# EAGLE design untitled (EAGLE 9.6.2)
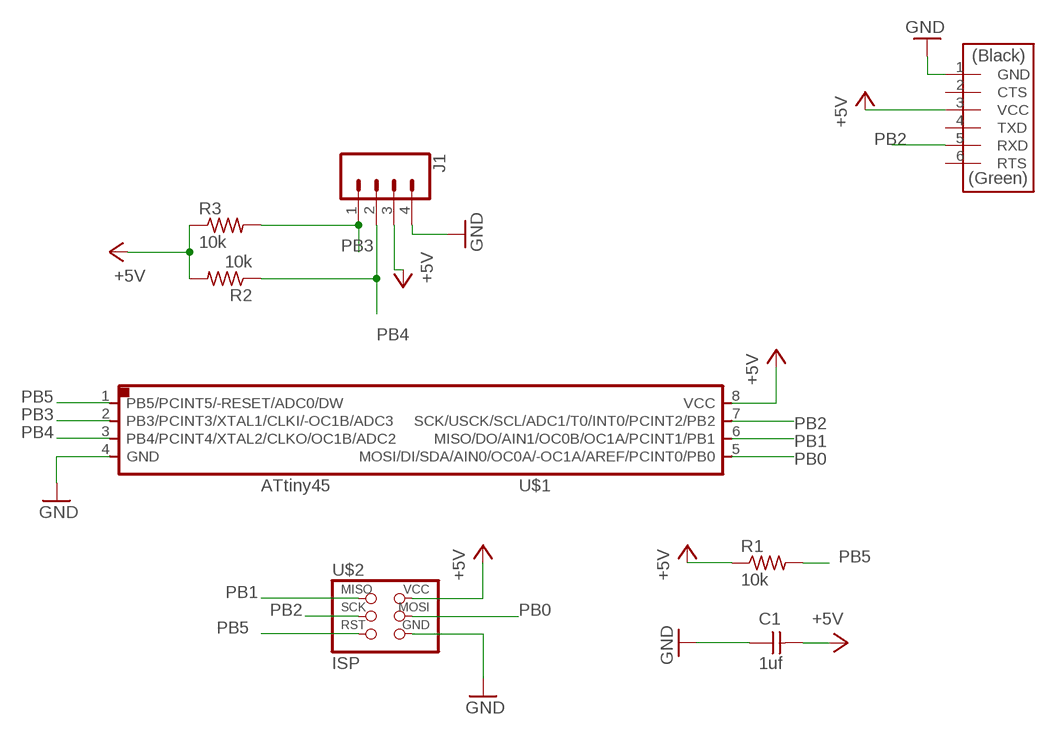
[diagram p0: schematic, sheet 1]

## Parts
C1  1uf  CAP_UNPOLARIZEDFAB  [C1206FAB]
J1  CONN_04LONGPADS  [1X04_LONGPADS]
R1  10k  R1206FAB  [R1206FAB]
R2  10k  R1206FAB  [R1206FAB]
R3  10k  R1206FAB  [R1206FAB]
U$1  ATTINY45  UC_ATTINY45SI  [SOIC8]
U$2  ISP  CONN_03X2_AVRISPSMD  [2X03SMD]
U$3  CONN_06_FTDI-SMD-HEADER  [1X06SMD]

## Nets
+5V: C1.2 J1.3 R1.1 R2.2 R3.1 U$1.8(VCC) U$2.2(VCC) U$3.3(VCC)
GND: C1.1 J1.4 U$1.4(GND) U$2.6(GND) U$3.1(GND)
PB0: U$1.5(MOSI/DI/SDA/AIN0/OC0A/-OC1A/AREF/PCINT0/PB0) U$2.4(MOSI)
PB1: U$1.6(MISO/DO/AIN1/OC0B/OC1A/PCINT1/PB1) U$2.1(MISO)
PB2: U$1.7(SCK/USCK/SCL/ADC1/T0/INT0/PCINT2/PB2) U$2.3(SCK) U$3.5(RXD)
PB3: J1.1 R3.2 U$1.2(PB3/PCINT3/XTAL1/CLKI/-OC1B/ADC3)
PB4: J1.2 R2.1 U$1.3(PB4/PCINT4/XTAL2/CLKO/OC1B/ADC2)
PB5: R1.2 U$1.1(PB5/PCINT5/-RESET/ADC0/DW) U$2.5(RST)
Unconnected: U$3.2(CTS) U$3.4(TXD) U$3.6(RTS)

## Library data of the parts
C1 = fab:CAP_UNPOLARIZED
J1 = SparkFun-Connectors:CONN_04: Multi connection point. Often used as Generic Header-pin footprint for 0.1 inch spaced/style header connections On any of the 0.1 inch spaced packages, you can populate with these: Break Away Headers - Straight (PRT-00116) Break Away Male Headers - Right Angle (PRT-00553) Female Headers (PRT-00115)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; PROD_ID: CONN-09696
R1-R3 = fab:R: Resistor (US Symbol)
U$1 = fab:UC_ATTINY45
U$2 = fab:CONN_03X2_AVRISP
U$3 = fab:CONN_06_FTDI-SMD-HEADER

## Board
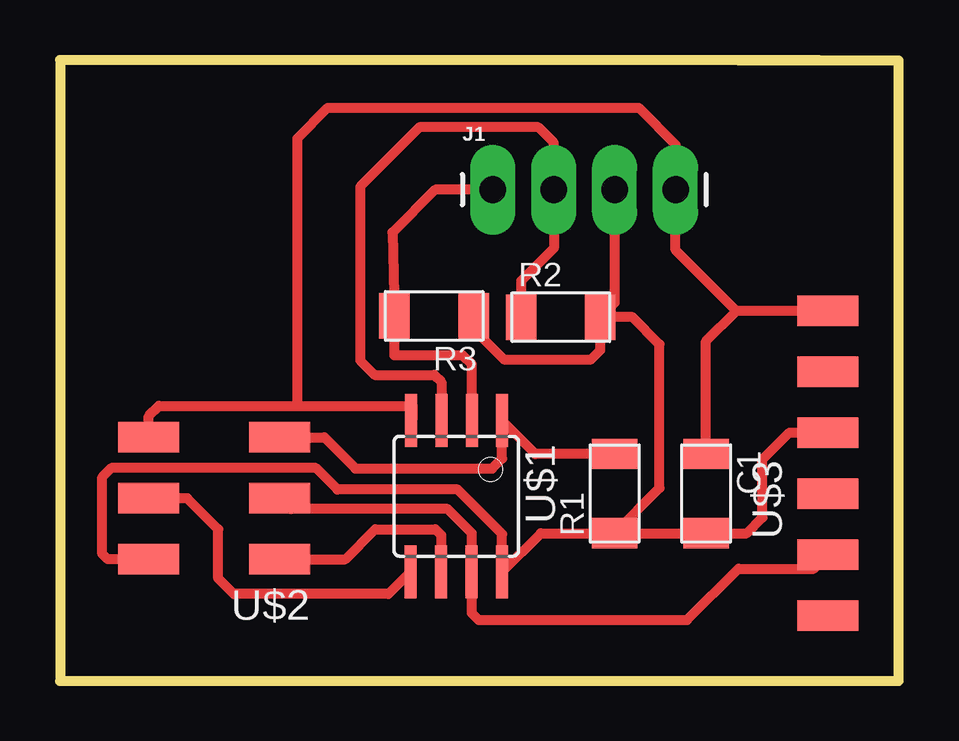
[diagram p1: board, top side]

Size 34.97 x 25.9 mm. Coordinates in mm from the lower left corner, seen from the top.
Outline: 31.63,25.9 0,25.9 0,0 34.97,0 34.97,25.87 28.28,25.87
Copper layers (1*16): Top 0.035mm / dielectric 1.5mm / Bottom 0.035mm
Design rules "default *": minimum track width 6mil, minimum drill 0.35mm, track to track 16mil, track to pad 16mil, pad to pad 16mil, via to via 16mil, smd to smd 16mil, copper to edge 40mil, drill to drill 6mil, minimum pad ring 10mil, minimum via ring 8mil, stop-mask expansion 4mil, vias tented up to drill 0mil, thermal gap 10mil

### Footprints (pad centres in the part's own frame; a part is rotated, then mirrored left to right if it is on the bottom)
C1206FAB = smd 1.27 x 1.905: 1 -1.651,0; 2 1.651,0
1X04_LONGPADS = drill 1.118 pad 1.88 long: 1 0,0; 2 2.54,0; 3 5.08,0; 4 7.62,0
R1206FAB = smd 1.27 x 1.905: 1 -1.651,0; 2 1.651,0
SOIC8 = smd 0.5 x 2.2: 1 -1.905,-3.154; 2 -0.645,-3.154; 3 0.625,-3.154; 4 1.895,-3.154; 5 1.905,3.154; 6 0.635,3.154; 7 -0.635,3.154; 8 -1.905,3.154
2X03SMD = smd 2.54 x 1.27: 1 -2.54,2.54; 2 2.92,2.54; 3 -2.54,0; 4 2.92,0; 5 -2.54,-2.54; 6 2.92,-2.54
1X06SMD = smd 2.54 x 1.27: 1 0,6.35; 2 0,3.81; 3 0,1.27; 4 0,-1.27; 5 0,-3.81; 6 0,-6.35

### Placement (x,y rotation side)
C1  26.93,7.82 270 top
J1  18.04,20.49 0 top
R1  23.12,7.82 90 top
R2  20.88,15.17 0 top
R3  15.6,15.22 180 top
U$1  16.52,7.71 180 top
U$2  6.63,7.62 180 top
U$3  32.01,9.09 0 top

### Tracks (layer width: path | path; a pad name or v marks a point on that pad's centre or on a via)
+5V
  Top 0.406: U$3.3 30.41,10.36 29.28,9.23 29.28,6.82 28.63,6.17 C1.2 R1.1 | R1.1 20.04,6.17 U$1.8 18.43,6.13 16.58,7.98 11.57,7.98 10.67,8.88 2.14,8.88 1.77,8.51 1.77,5.3 1.99,5.08 U$2.2 | R2.2 23.12,15.77 J1.3 | R3.1 17.25,14.67 18.5,13.41 22.14,13.41 22.53,13.8 R2.2 | R1.1 25,8.04 25,14.04 23.87,15.17 R2.2
GND
  Top 0.406: C1.1 26.93,14.17 28.2,15.44 | U$3.1 28.2,15.44 | 28.2,15.44 25.66,17.98 J1.4 25.66,22.36 24.13,23.9 11.17,23.9 9.9,22.63 9.9,11.47 | U$2.6 3.71,11.05 4.13,11.47 9.9,11.47 | 9.9,11.47 14.7,11.47 14.7,10.93 U$1.4
PB0
  Top 0.406: U$1.5 13.7,3.63 7.25,3.63 6.6,4.28 6.6,6.32 5.3,7.62 U$2.4
PB1
  Top 0.406: U$2.1 11.9,5.08 13.14,6.32 15.65,6.32 15.89,6.08 U$1.6
PB2
  Top 0.406: U$3.5 31.42,4.68 28.28,4.68 26.14,2.54 17.45,2.54 17.16,2.83 U$1.7 17.16,6.17 16.16,7.17 9.62,7.17 U$2.3
PB3
  Top 0.406: J1.1 15.64,20.49 13.86,18.71 R3.2 13.95,13.58 16.8,13.58 17.17,13.21 U$1.2
PB4
  Top 0.406: R2.1 19.22,16.68 20.58,18.04 J1.2 20.58,22.44 19.94,23.08 14.99,23.08 12.51,20.61 12.51,13.37 13.12,12.76 15.6,12.76 15.9,12.47 U$1.3
PB5
  Top 0.406: R1.2 19.82,9.47 U$1.1 18.43,9.27 18.02,8.86 12.31,8.86 11.02,10.16 U$2.5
